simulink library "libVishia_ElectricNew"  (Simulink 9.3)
settings: Solver=ode3  StartTime=0.0  StopTime=1  FixedStep=0.02/16384  RelTol=1e-3
undefined symbols (not defined in the file or in its folder): bool2single, hi, lib_Conv, lo, Rps
libraries: fl_lib x4, ee_lib x4, nesl_utility x2

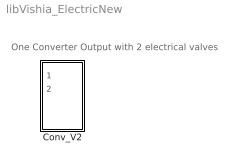
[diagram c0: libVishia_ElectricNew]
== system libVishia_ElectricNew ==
  note: One Converter Output with 2 electrical valves
  Conv_V2 : Subsystem

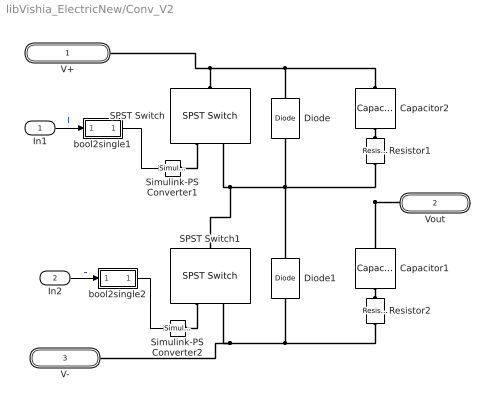
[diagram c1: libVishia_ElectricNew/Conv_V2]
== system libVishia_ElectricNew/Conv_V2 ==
  In1 : Inport
  In2 : Inport  Port=2
  Capacitor1 : fl_lib/Electrical/Electrical Elements/Capacitor  c=Cp nF  r=0 Ohm  g=0 1/Ohm  i_specify=off  i_priority=None  i=0 A  i_nominal_specify=off  i_nominal_unit=A  i_nominal_value=1  v_specify=off  v_priority=None  v=0 V  v_nominal_specify=off  v_nominal_unit=V  v_nominal_value=1  vc_specify=off  vc_priority=High  vc=0 V  vc_nominal_specify=off  vc_nominal_unit=V  vc_nominal_value=1
  Capacitor2 : fl_lib/Electrical/Electrical Elements/Capacitor  c=Cp nF  r=0 Ohm  g=0 1/Ohm  i_specify=off  i_priority=None  i=0 A  i_nominal_specify=off  i_nominal_unit=A  i_nominal_value=1  v_specify=off  v_priority=None  v=0 V  v_nominal_specify=off  v_nominal_unit=V  v_nominal_value=1  vc_specify=off  vc_priority=High  vc=0 V  vc_nominal_specify=off  vc_nominal_unit=V  vc_nominal_value=1
  Diode : ee_lib/Semiconductors & Converters/Diode  ModelType=ee.enum.diode.modelType.pwl  Vf=0.6 V  Ron=0.01 Ohm  Goff=1e-8 S  prmExp=ee.enum.diode.expParam.useTwo  I12=[.0137, .545] A  V12=[.6, .7] V  IS=1e-12 A  ec=1  I1=0.0137 A  V1=0.6 V  RS=0 Ohm  Tmeas=25 degC  N_series=1  N_parallel=1  Rz=0.3 Ohm  BV=inf V  C_param=ee.enum.diode.capParam.fixed  CJ=5 pF  CJ0=5 pF  VJ=1 V  Mgrad=0.5  Vvec=[.1, 10, 100] V  Cvec=[3.5, 1, .4] pF  FC=0.5  Q_param=ee.enum.diode.recoveryParam.off  iRM=-7.15 A  iF=4 A  didt=-750 A/us  trr_factor=3  trr=115 ns  Qrr=1500 s*uA  TT=50 ns  tau=100 ns  T_param=ee.enum.diode.temperatureParam.off  IS_T2=1.25e-7 A  I1_T2=0.245 A  V1_T2=0.5 V  Tmeas2=125 degC  EG_param=ee.enum.diode.egapParam.material_si  EG=1.11 eV  XTI_param=ee.enum.diode.xtiParam.pn  XTI=3  dBVdT=0 V/K  Tdevice=25 degC  i_specify=off  i_priority=None  i=0 A  i_nominal_specify=off  i_nominal_unit=A  i_nominal_value=1  v_specify=off  v_priority=None  v=0 V  v_nominal_specify=off  v_nominal_unit=V  v_nominal_value=1  i_capacitor_specify=off  i_capacitor_priority=None  i_capacitor=0 A  i_capacitor_nominal_specify=off  i_capacitor_nominal_unit=A  i_capacitor_nominal_value=1  v_capacitor_specify=off  v_capacitor_priority=None  v_capacitor=0 V  v_capacitor_nominal_specify=off  v_capacitor_nominal_unit=V  v_capacitor_nominal_value=1  power_dissipated_specify=off  power_dissipated_priority=None  power_dissipated=0 W  power_dissipated_nominal_specify=off  power_dissipated_nominal_unit=W  power_dissipated_nominal_value=1  Rth=[0, 10] K/W  thermal_mass_parameterization=ee.enum.thermalNetwork.timeconstant  thermal_mass=[0, 1] J/K  thermal_time_constant=[0, 10] s  thermal_mass_initial_temperatures=[25, 25] degC
  Diode1 : ee_lib/Semiconductors & Converters/Diode  ModelType=ee.enum.diode.modelType.pwl  Vf=0.6 V  Ron=0.01 Ohm  Goff=1e-8 S  prmExp=ee.enum.diode.expParam.useTwo  I12=[.0137, .545] A  V12=[.6, .7] V  IS=1e-12 A  ec=1  I1=0.0137 A  V1=0.6 V  RS=0 Ohm  Tmeas=25 degC  N_series=1  N_parallel=1  Rz=0.3 Ohm  BV=inf V  C_param=ee.enum.diode.capParam.fixed  CJ=5 pF  CJ0=5 pF  VJ=1 V  Mgrad=0.5  Vvec=[.1, 10, 100] V  Cvec=[3.5, 1, .4] pF  FC=0.5  Q_param=ee.enum.diode.recoveryParam.off  iRM=-7.15 A  iF=4 A  didt=-750 A/us  trr_factor=3  trr=115 ns  Qrr=1500 s*uA  TT=50 ns  tau=100 ns  T_param=ee.enum.diode.temperatureParam.off  IS_T2=1.25e-7 A  I1_T2=0.245 A  V1_T2=0.5 V  Tmeas2=125 degC  EG_param=ee.enum.diode.egapParam.material_si  EG=1.11 eV  XTI_param=ee.enum.diode.xtiParam.pn  XTI=3  dBVdT=0 V/K  Tdevice=25 degC  i_specify=off  i_priority=None  i=0 A  i_nominal_specify=off  i_nominal_unit=A  i_nominal_value=1  v_specify=off  v_priority=None  v=0 V  v_nominal_specify=off  v_nominal_unit=V  v_nominal_value=1  i_capacitor_specify=off  i_capacitor_priority=None  i_capacitor=0 A  i_capacitor_nominal_specify=off  i_capacitor_nominal_unit=A  i_capacitor_nominal_value=1  v_capacitor_specify=off  v_capacitor_priority=None  v_capacitor=0 V  v_capacitor_nominal_specify=off  v_capacitor_nominal_unit=V  v_capacitor_nominal_value=1  power_dissipated_specify=off  power_dissipated_priority=None  power_dissipated=0 W  power_dissipated_nominal_specify=off  power_dissipated_nominal_unit=W  power_dissipated_nominal_value=1  Rth=[0, 10] K/W  thermal_mass_parameterization=ee.enum.thermalNetwork.timeconstant  thermal_mass=[0, 1] J/K  thermal_time_constant=[0, 10] s  thermal_mass_initial_temperatures=[25, 25] degC
  Resistor1 : fl_lib/Electrical/Electrical Elements/Resistor  R=Rps Ohm  i_specify=off  i_priority=None  i=0 A  i_nominal_specify=off  i_nominal_unit=A  i_nominal_value=1  v_specify=off  v_priority=None  v=0 V  v_nominal_specify=off  v_nominal_unit=V  v_nominal_value=1
  Resistor2 : fl_lib/Electrical/Electrical Elements/Resistor  R=Rps Ohm  i_specify=off  i_priority=None  i=0 A  i_nominal_specify=off  i_nominal_unit=A  i_nominal_value=1  v_specify=off  v_priority=None  v=0 V  v_nominal_specify=off  v_nominal_unit=V  v_nominal_value=1
  SPST Switch : ee_lib/Switches & Breakers/SPST Switch  R_closed=0.01 Ohm  G_open=1e-6 S  Threshold=0 V  Width=0 V  model_dynamics=0  t_on=1e-3 s  t_off=1e-3 s  initial_vT=0 V
  SPST Switch1 : ee_lib/Switches & Breakers/SPST Switch  R_closed=0.01 Ohm  G_open=1e-6 S  Threshold=0 V  Width=0 V  model_dynamics=0  t_on=1e-3 s  t_off=1e-3 s  initial_vT=0 V
  Simulink-PS Converter1 : nesl_utility/Simulink-PS Converter  PhysicalDomain=network_engine_domain  SubClassName=ps_input  LeftPortType=input  RightPortType=output  PseudoPeriodic=off  Frequencies=[]  NoiseDistribution=none  NoiseParameters=[]  Unit=1  AffineConversion=off  FilteringAndDerivatives=provide  SimscapeFilterOrder=1  InputFilterTimeConstant=0.001  UdotUserProvided=0
  Simulink-PS Converter2 : nesl_utility/Simulink-PS Converter  PhysicalDomain=network_engine_domain  SubClassName=ps_input  LeftPortType=input  RightPortType=output  PseudoPeriodic=off  Frequencies=[]  NoiseDistribution=none  NoiseParameters=[]  Unit=1  AffineConversion=off  FilteringAndDerivatives=provide  SimscapeFilterOrder=1  InputFilterTimeConstant=0.001  UdotUserProvided=0
  bool2single1 : Subsystem  AncestorBlock=lib_Conv/bool2single
  bool2single2 : Subsystem  AncestorBlock=lib_Conv/bool2single
  V+ : PMIOPort  Side=Left
  Vout : PMIOPort  Port=2  Side=Right
  V- : PMIOPort  Port=3  Side=Left
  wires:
  bool2single2/1(y) -> Simulink-PS Converter2/1
  bool2single1/1(y) -> Simulink-PS Converter1/1
  In2/1 -> bool2single2/1(b)  "L"
  In1/1 -> bool2single1/1(b)  "H"
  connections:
  Resistor1/RConn1 -- Diode/LConn1 -- Diode1/RConn1 -- SPST Switch1/RConn1 -- SPST Switch/LConn2 -- Capacitor1/LConn1 -- Vout/RConn1
  Resistor2/RConn1 -- Diode1/LConn1 -- V-/RConn1 -- SPST Switch1/LConn2
  Resistor2/LConn1 -- Capacitor1/RConn1
  SPST Switch1/LConn1 -- Simulink-PS Converter2/RConn1
  Capacitor2/LConn1 -- Diode/RConn1 -- V+/RConn1 -- SPST Switch/RConn1
  SPST Switch/LConn1 -- Simulink-PS Converter1/RConn1
  Resistor1/LConn1 -- Capacitor2/RConn1

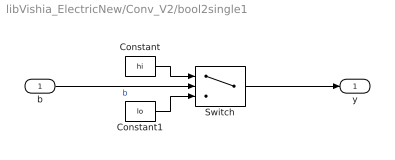
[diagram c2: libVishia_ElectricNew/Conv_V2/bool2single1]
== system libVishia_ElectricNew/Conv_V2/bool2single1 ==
  b : Inport
  Constant : Constant  Value=hi  OutDataTypeStr=double
  Constant1 : Constant  Value=lo  OutDataTypeStr=double
  Switch : Switch  Criteria=u2 ~= 0
  y : Outport  OutDataTypeStr=double
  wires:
  Switch/1 -> y/1
  b/1 -> Switch/2  "b"
  Constant1/1 -> Switch/3
  Constant/1 -> Switch/1

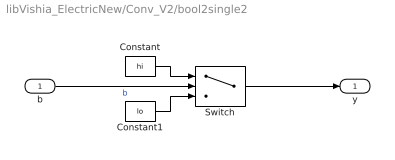
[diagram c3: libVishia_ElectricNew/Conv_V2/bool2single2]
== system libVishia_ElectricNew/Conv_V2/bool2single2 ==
  b : Inport
  Constant : Constant  Value=hi  OutDataTypeStr=double
  Constant1 : Constant  Value=lo  OutDataTypeStr=double
  Switch : Switch  Criteria=u2 ~= 0
  y : Outport  OutDataTypeStr=double
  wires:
  Switch/1 -> y/1
  b/1 -> Switch/2  "b"
  Constant1/1 -> Switch/3
  Constant/1 -> Switch/1
